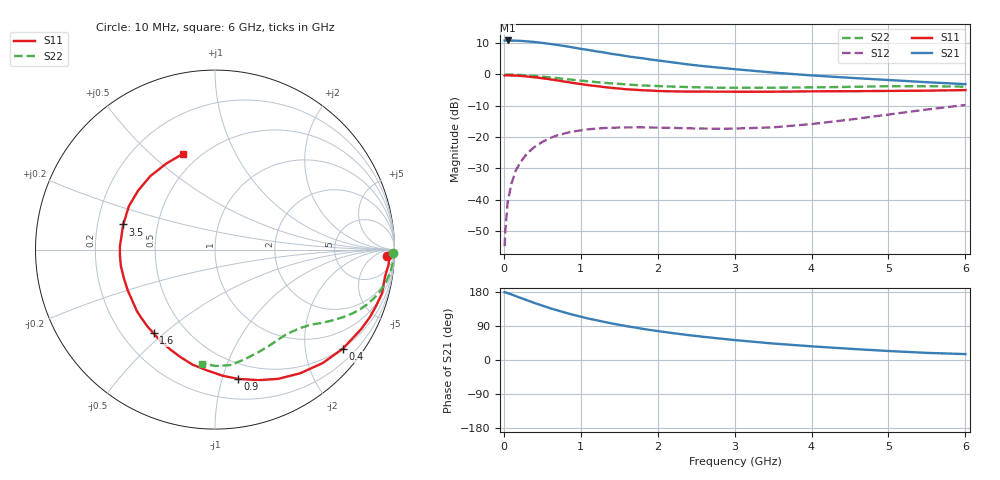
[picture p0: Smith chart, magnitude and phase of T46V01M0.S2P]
! Infineon Technologies  Discrete & RF Semiconductors
! BFR182T
! Si NPN RF Bipolar Junction Transistor in SC75
! VCE = 6 V  IC = 1 mA
! Common Emitter S-Parameters:  October  1999
# GHz  S  MA  R  50
!  f  S11  S21  S12  S22
! GHz  MAG  ANG  MAG  ANG  MAG  ANG  MAG  ANG
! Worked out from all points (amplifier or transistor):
!   36 points, 10 MHz to 6 GHz, reference 50 ohm
!   highest |S21| = 10.9 dB at 50 MHz (marker M1)
!   |S21| within 3 dB of that: start of sweep to 1.091 GHz
!   unconditionally stable (mu >= 1): 2.42 GHz to 4.592 GHz
!   at 250 MHz: K = 0.10, MSG = 18.8 dB, |S12| = -26.9 dB
!   at 1.4 GHz: K = 0.57, MSG = 11.8 dB, |S12| = -17.0 dB
!   at 6 GHz: K = 0.83, MSG = 3.3 dB, |S12| = -9.7 dB
!   S11 on the Smith chart (normalised r, x): 10 MHz: 28, -23; 400 MHz: 0.48, -2.85; 900 MHz: 0.36, -1.13; 1.6 GHz: 0.33, -0.46; 3.5 GHz: 0.31, +0.12; 6 GHz: 0.41, +0.64
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0.01  0.958 -2.0  3.475 178.7  0.0018 75.0  0.9911 -1.2
0.02  0.9756 -0.7  3.488 178.8  0.0033 97.4  0.9909 -0.7
0.05  0.9706 -5.0  3.496 176.3  0.0092 88.0  0.9971 -1.9
0.1  0.9591 -9.1  3.466 173.0  0.0181 86.5  0.9948 -3.8
0.15  0.9622 -14.6  3.474 169.0  0.0281 80.9  0.9896 -5.6
0.25  0.9414 -23.6  3.423 161.5  0.0451 75.6  0.9764 -9.2
0.4  0.9013 -37.8  3.304 150.3  0.0697 68.1  0.9482 -14.3
0.5  0.8712 -46.6  3.195 143.5  0.0833 63.1  0.9243 -17.2
0.6  0.8368 -55.4  3.077 136.8  0.0962 58.6  0.8992 -20.0
0.7  0.8017 -63.9  2.957 130.7  0.1069 54.5  0.8722 -22.5
0.8  0.7667 -71.6  2.836 124.9  0.1151 50.7  0.8457 -24.8
0.9  0.7318 -79.8  2.699 119.4  0.1222 47.3  0.8202 -26.8
1.1  0.6734 -94.1  2.466 109.3  0.1331 41.8  0.7754 -30.2
1.4  0.6102 -113.9  2.135 96.7  0.1406 35.5  0.7215 -34.5
1.6  0.5783 -126.3  1.957 89.1  0.1426 32.8  0.6922 -36.8
1.9  0.5536 -141.9  1.738 79.3  0.1417 30.7  0.6603 -40.5
2.2  0.5367 -154.9  1.557 70.8  0.1399 30.4  0.6395 -43.8
2.8  0.5308 -176.2  1.284 56.8  0.1356 34.7  0.6144 -51.7
3.5  0.5302 164.7  1.072 43.5  0.1428 45.2  0.6149 -60.7
4.5  0.54 142.5  0.884 29.6  0.19 58.1  0.6336 -75.1
5.5  0.5508 119.5  0.752 18.8  0.2752 60.4  0.6485 -89.6
6  0.5626 108.7  0.7 15.6  0.3255 58.1  0.6388 -96.5
